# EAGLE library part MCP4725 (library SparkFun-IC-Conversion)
MCP4725 DAC Microchip 12-bit I2C DAC, SOT23-6 Datasheet SparkFun Products SparkFun I2C DAC Breakout - MCP4725 (BOB-12918)
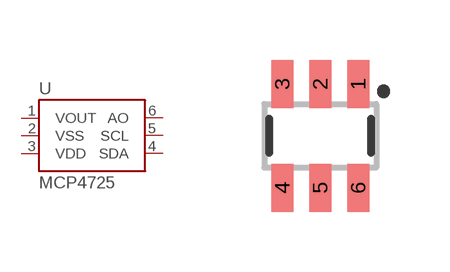
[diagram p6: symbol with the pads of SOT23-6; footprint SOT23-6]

Designator prefix U

## MCP4725SOT-23 (PROD_ID: IC-08886; VALUE: MCP4725)  [SOT23-6]
1  VOUT
2  VSS
3  VDD
4  SDA
5  SCL
6  AO

## Footprint SOT23-6 (pad centres in mm)
SOT23-6 Specifications: Pin count: 6 Example device(s): MCP4725
smd 0.55 x 1.2: 1 0.95,1.3; 2 0,1.3; 3 -0.95,1.3; 4 -0.95,-1.3; 5 0,-1.3; 6 0.95,-1.3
